FUNCTION_BLOCK FB18
TITLE =Set Motor Parameter
//*****************************************************************************
//* maxon motor ag
//* R&D
//* all rights reserved
//*****************************************************************************
//* Summary:  Set all motor parameters
//*
//* Remarks:
//*
//* Created under: STEP7 REV5.2+SP1
//*****************************************************************************
//* History:
//* 18.05.2004 | INA   first release
//*
//*
//*****************************************************************************
//

AUTHOR:INA
FAMILY:Configur
NAME:SMotPara
VERSION:00.01


VAR_INPUT

Write : BOOL //A rising edge start the command

  NodeID : BYTE //Adress of the maxon device

  MotorType : WORD //Kind of Motor

  ContinuousCurrent : WORD //Maximal Continuous Current

  PeakCurrent : WORD //Maximal Peak Current

  PolePair : BYTE //Number of Pole Pairs

  ThermalTimeConstant : WORD //Thermal Time Constant

END_VAR
VAR_OUTPUT
  Done : BOOL //Data valid flag is TRUE if data were available

  Err : BOOL //Error flag is TRUE if an Error has occured, see ErrNo for more details

  ErrNo : DINT //Contains detailed error information

END_VAR
VAR
  xEdgeMerker : BOOL //Edge Merker

  xEdgeFlag : BOOL //Edge Flag

  xStep : INT
END_VAR

BEGIN

NETWORK
TITLE = Activate the service function
//

// SDO Write "Set Motor Parameter"

       U    #Write
       FP   #xEdgeFlag                   // recognize a positiv edge of the Read signal
       =    #xEdgeMerker                 // and set the xEdgeMerker for one cycle to true

       L    #xStep
       L    0
       ==I
       U    #xEdgeMerker
       SPB  nstp                         // iStep = 1 -> fnc1

       L    #xStep                       // jump list
       SPL  List
       SPA  rdef
       SPA  fnc1
       SPA  fncE
List  :SPA  rdef

rdef  :NOP  0
       R    #Done                        // reset Done
       R    #Err
       L    0
       T    #xStep                       // iStep = 0
       SPA  end

fnc1  :NOP  0
       CALL FC15
         NodeID:=#NodeID
         Index:=DW#16#00006402
         SubIndex:=DW#16#00000000
         ValueIn:=#MotorType
         RET_VAL:=#Done
         Err:=#Err
         ErrNo:=#ErrNo

       L    1
       U    #Err
       SPB  fncE

       NOP  0
       CALL FC15
         NodeID:=#NodeID
         Index:=DW#16#00006410
         SubIndex:=DW#16#00000001
         ValueIn:=#ContinuousCurrent
         RET_VAL:=#Done
         Err:=#Err
         ErrNo:=#ErrNo

       L    1
       U    #Err
       SPB  fncE

       NOP  0
       CALL FC15
         NodeID:=#NodeID
         Index:=DW#16#00006410
         SubIndex:=DW#16#00000002
         ValueIn:=#PeakCurrent
         RET_VAL:=#Done
         Err:=#Err
         ErrNo:=#ErrNo

       L    1
       U    #Err
       SPB  fncE

       NOP  0
       CALL FC14
         NodeID:=#NodeID
         Index:=DW#16#00006410
         SubIndex:=DW#16#00000003
         ValueIn:=#PolePair
         RET_VAL:=#Done
         Err:=#Err
         ErrNo:=#ErrNo

       L    1
       U    #Err
       SPB  fncE

       NOP  0
       CALL FC15
         NodeID:=#NodeID
         Index:=DW#16#00006410
         SubIndex:=DW#16#00000005
         ValueIn:=#MotorType
         RET_VAL:=#Done
         Err:=#Err
         ErrNo:=#ErrNo

fncE  :NOP  0
       L    0
       T    #xStep
       SPA  end

nstp  :NOP  0
       L    #xStep
       INC            1
       T    #xStep

end   :NOP  0
END_FUNCTION_BLOCK
